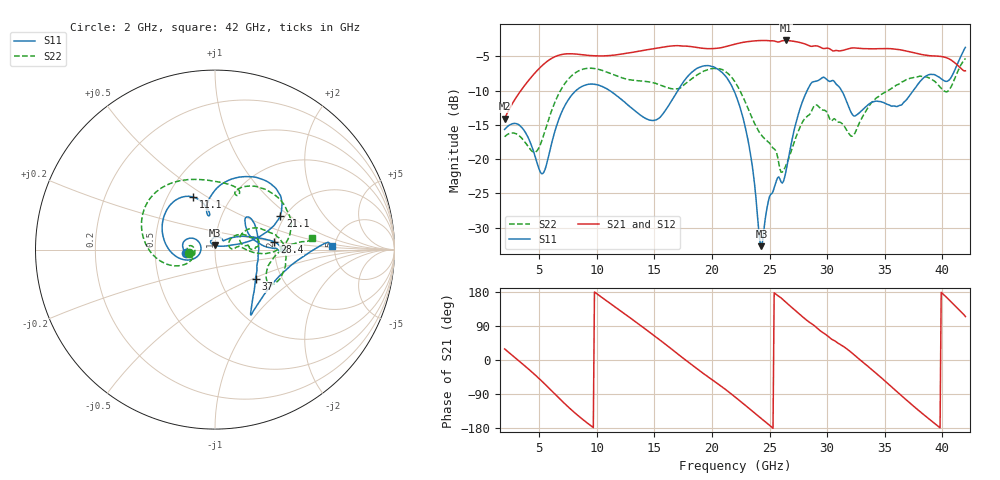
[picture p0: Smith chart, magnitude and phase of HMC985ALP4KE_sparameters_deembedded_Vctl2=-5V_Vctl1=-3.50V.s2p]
!s2p File: Measurements: S11, S21, S12, S22
# GHz S dB R 50.0
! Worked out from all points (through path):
!   401 points, 2 GHz to 42 GHz, reference 50 ohm
!   highest |S21| = -2.69 dB at 26.4 GHz (marker M1); lowest = -14.1 dB at 2 GHz (marker M2)
!   lowest |S11| = -32.7 dB at 24.3 GHz (marker M3), VSWR 1.05, Z = 50.1 + j2.32 ohm
!   |S11| at or under -10 dB: start of sweep to 8.194 GHz; 21.91 GHz to 28.26 GHz (6.357 GHz wide, 25.3 % of centre); 31.26 GHz to 37.47 GHz (6.215 GHz wide, 18.1 % of centre)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
!   |S22| runs from -21.9 to -5.3 dB; largest |S21 - S12| = 0.00063
!   S11 on the Smith chart (normalised r, x): 2 GHz: 0.72, -0.02; 11.1 GHz: 0.67, +0.44; 21.1 GHz: 1.88, +0.86; 28.4 GHz: 1.98, +0.19; 37 GHz: 1.48, -0.52; 42 GHz: 4.74, +0.36
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2  -15.66 -174.2  -14.10 29.3  -14.11 29.3  -16.72 -172.8
3.5  -15.39 160.6  -9.79 -9.0  -9.79 -9.0  -16.96 171.1
5.3  -22.11 179.5  -6.28 -57.8  -6.29 -57.8  -16.95 -156.6
6.9  -13.35 -168.7  -4.75 -105.9  -4.75 -105.9  -9.84 -170.3
8.7  -9.41 147.4  -4.76 -154.8  -4.76 -154.8  -6.93 152.8
11.1  -9.97 112.7  -4.89 150.7  -4.89 150.7  -7.45 114.2
13.4  -13.05 99.6  -4.33 100.1  -4.33 100.1  -8.52 82.7
15.4  -14.04 102.2  -3.75 54.6  -3.76 54.6  -9.12 67.0
17.9  -7.91 77.1  -3.53 -4.7  -3.53 -4.7  -8.73 68.5
21.1  -7.75 27.6  -3.62 -76.0  -3.62 -76.0  -7.15 15.6
22  -10.35 18.8  -3.23 -97.4  -3.23 -97.4  -8.73 1.5
23.2  -17.85 13.5  -2.84 -127.2  -2.84 -127.2  -12.88 -4.6
24.3  -32.69 85.2  -2.69 -154.7  -2.69 -154.6  -16.51 4.9
25  -25.45 117.0  -2.73 -172.4  -2.73 -172.4  -17.66 7.5
26.4  -21.98 43.1  -2.69 152.9  -2.69 152.9  -21.01 28.6
28.4  -9.53 7.4  -3.42 100.9  -3.42 100.9  -13.58 18.8
28.7  -8.77 2.4  -3.54 94.8  -3.54 94.8  -12.77 17.4
32.4  -13.72 28.2  -3.78 12.0  -3.78 12.0  -16.23 26.2
35.4  -12.10 15.0  -3.88 -65.6  -3.88 -65.6  -9.89 17.3
37  -11.09 -35.8  -4.27 -108.7  -4.27 -108.7  -8.33 3.9
39.7  -8.02 -55.9  -4.99 -176.4  -4.99 -176.4  -9.29 -31.8
42  -3.69 1.9  -7.11 114.6  -7.11 114.6  -5.31 7.0
